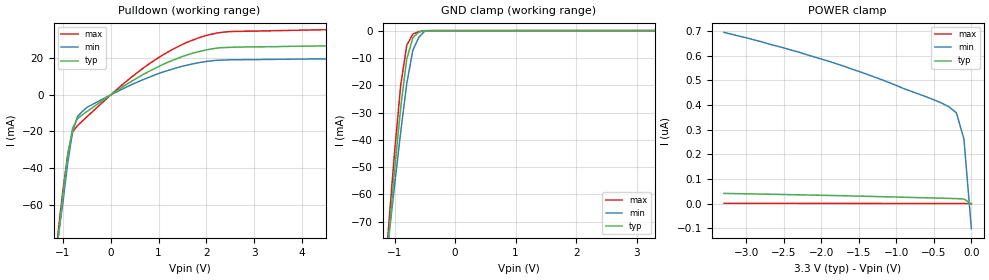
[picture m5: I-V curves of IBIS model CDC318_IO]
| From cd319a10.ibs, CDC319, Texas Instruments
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|   Model CDC318_IO
[Model]   CDC318_IO
Model_type   I/O_open_drain
Polarity   Non-Inverting
Vinl = 0.99V
Vinh = 2.31V
Vmeas = 1.5V
Cref = 400pF
Rref = 1000
Vref = 3.3
|   variable   typ   min   max
C_comp   6.2p   NA   NA
[Voltage range]   3.3   3.135   3.465
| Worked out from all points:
|   slope of the pulldown table from 0 to 0.495 V, typ, clamps not added: 59.4 ohm
|   GND clamp passes 1 mA (typ) near -0.62 V on its own axis
[Pulldown]
|  Voltage   I(typ)   I(min)   I(max)
-3.3V     -671mA     -564mA     -793mA
-1.2V     -102mA     -97.1mA    -103mA
-1.1V     -77mA      -77.5mA    -73.8mA
-1V       -53.3mA    -58mA      -51.5mA
-900mV    -32.6mA    -36.7mA    -32mA
-800mV    -18.2mA    -20.1mA    -20.2mA
-700mV    -13.1mA    -11.9mA    -16.9mA
-500mV    -9.14mA    -6.88mA    -12mA
700mV     11.4mA     8.53mA     15mA
1.6V      21.8mA     16.2mA     28.7mA
2.5V      25.9mA     19.1mA     34.5mA
6.6V      27.4mA     20.1mA     36.4mA
[GND_Clamp]
|  Voltage   I(typ)   I(min)   I(max)
-3.3V     -672mA     -565mA     -794mA
-1.2V     -101mA     -96.6mA    -102mA
-1.1V     -75.4mA    -76.3mA    -71.7mA
-1V       -50.8mA    -56.3mA    -44mA
-900mV    -28.1mA    -37.1mA    -20mA
-800mV    -10.4mA    -19.4mA    -5.36mA
-700mV    -2.63mA    -7.24mA    -1.32mA
-600mV    -569uA     -2.42mA    -333uA
-500mV    -49.5uA    -180uA     -39.5uA
3.3V      16.2pA     357nA      -499nA
[POWER_clamp]
|  Voltage   I(typ)   I(min)   I(max)
-3.3V     41.7nA     694nA      1.69nA
-2.3V     36.1nA     614nA      1.4nA
-1.7V     32.2nA     557nA      1.21nA
-600mV    24nA       433nA      845pA
-300mV    21.6nA     393nA      742pA
-200mV    20.7nA     368nA      703pA
-100mV    19.1nA     263nA      661pA
0V        16.2pA     -101nA     408pA
[Ramp]
|  variable   typ   min   max
dV/dt_f   1.32/140n   1.25/200n   1.39/90n   | internal slope
dV/dt_r   1.32/1n   1.25/1n   1.39/1n   | internal slope
